PROGRAM MAIN
VAR
	S0: BOOL;
	S1: BOOL;
	L0: BOOL;
	p12_controlLight_instance: p12_controlLight;
END_VAR

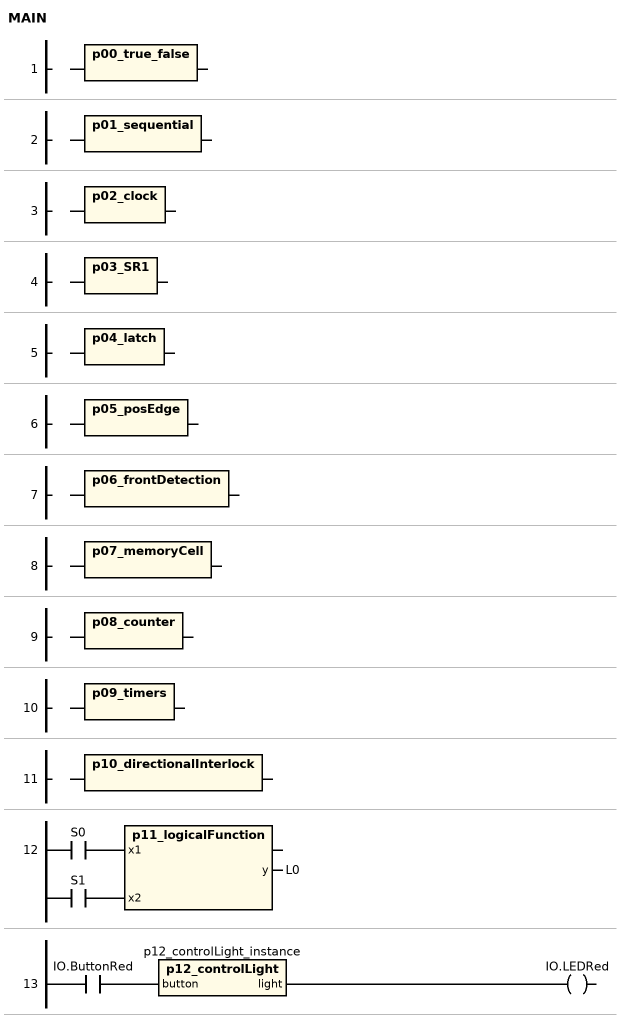
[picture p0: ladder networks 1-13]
// NETWORK 1
p00_true_false();

// NETWORK 2
p01_sequential();

// NETWORK 3
p02_clock();

// NETWORK 4
p03_SR1();

// NETWORK 5
p04_latch();

// NETWORK 6
p05_posEdge();

// NETWORK 7
p06_frontDetection();

// NETWORK 8
p07_memoryCell();

// NETWORK 9
p08_counter();

// NETWORK 10
p09_timers();

// NETWORK 11
p10_directionalInterlock();

// NETWORK 12
p11_logicalFunction(x1 := S0, x2 := S1, y => L0);

// NETWORK 13
p12_controlLight_instance(button := IO.ButtonRed); // p12_controlLight
IO.LEDRed := p12_controlLight_instance.light;

END_PROGRAM
